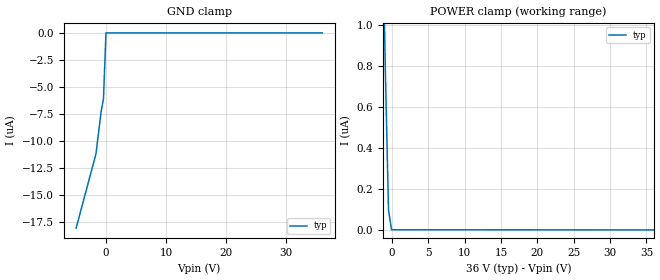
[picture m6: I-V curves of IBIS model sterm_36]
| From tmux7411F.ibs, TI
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| sterm_36
[Model]   sterm_36
Model_type   Terminator
|   typ   min   max
C_comp   4.014581e-12   NA   NA
[Voltage Range]   36   NA   NA
[Temperature Range]   27   NA   NA
[Power Clamp Reference]   36   NA   NA
[GND Clamp Reference]   0   NA   NA
[GND Clamp]
|   Voltage   I(typ)   I(min)   I(max)
-5V       -18.11uA   NA         NA
-1.687V   -11.19uA   NA         NA
-858.6mV  -7.391uA   NA         NA
-444.4mV  -6.095uA   NA         NA
-30.3mV   -851.9pA   NA         NA
36V       1.028nA    NA         NA
[POWER Clamp]
|   Voltage   I(typ)   I(min)   I(max)
-5V       8.865uA    NA         NA
-1.273V   1.509uA    NA         NA
-858.6mV  745.1nA    NA         NA
-444.4mV  96.07nA    NA         NA
-30.3mV   1.046nA    NA         NA
36V       -427.2pA   NA         NA
